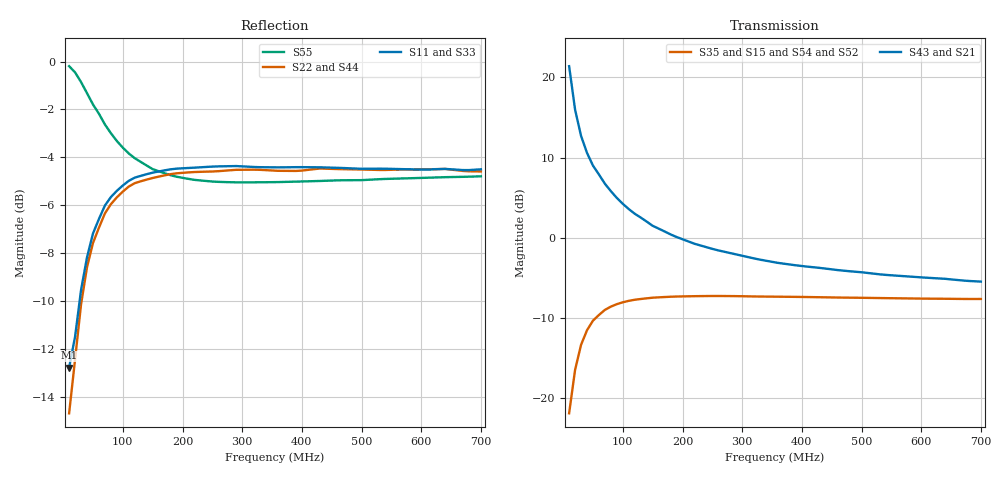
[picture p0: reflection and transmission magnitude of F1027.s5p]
! Date: Fri Jul 21 10:18:01 1995
!  POLYFET RF DEVICES
!  F1027 (Each Side)
!  S PARAMETERS
!  VDS=28V, IDQ=1.20mA
!AWR Design Environment (2053) Wed Feb 04 14:30:54 2004
!freq-unit  param-type  data-format  keyword  impedance-ohms
# MHz  S  MA  R  50
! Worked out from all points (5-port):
!   70 points, 10 MHz to 700 MHz, reference 50 ohm
!   strongest paths, dB at 10 MHz, 180 MHz, 360 MHz, 530 MHz, 700 MHz:
!     S43: 21.4, 0.4, -3.1, -4.6, -5.5
!     S21: 21.4, 0.4, -3.1, -4.6, -5.5
!     S35: -21.9, -7.4, -7.4, -7.5, -7.6
!     S15: -21.9, -7.4, -7.4, -7.5, -7.6
!     S54: -22.0, -7.5, -7.4, -7.6, -7.7
!     S52: -22.0, -7.5, -7.4, -7.6, -7.7
!   lowest |S11| = -12.8 dB at 10 MHz (marker M1), VSWR 1.60, Z = 47.8 - j23 ohm
!   |S11| at or under -10 dB: start of sweep to 27.61 MHz
